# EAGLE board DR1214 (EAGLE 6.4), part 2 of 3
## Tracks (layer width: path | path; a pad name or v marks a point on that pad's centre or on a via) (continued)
GND  (via drill 0.15 layers 1-2, 0.15 layers 15-16, 0.25, 0.25 layers 2-15) (continued)
  other vias: 78.6,20.35 96.1,22.8 89.1,26 92.2,24.8 102,20.8 70,30 64.2,33.8 46.8,18.5 22.2,1.2 12.4,1.6 19.2,1.6 27.5,1.15 32,1.2 35.2,1.2 44,1.2 48.8,1.2 59.2,1.2 65.6,1.2 71.2,1.2 77.6,1.6 83.2,1.6 86,8.8 86.4,4 93.6,8.8 98.4,10.8 106.4,12.8 106.4,18.4 106.4,24.8 106.4,30.4 106.4,37.6 97.6,47.2 106.4,50 106.4,46.4 98.4,54 96,58.4 96,64 89.6,64 81.6,64 74.4,64 66.4,64 60,64 52.8,64 48,64 40.8,64 33.6,64 12.8,64 19.2,64 26.4,64 11.2,56 9.6,54.4 3.2,52.8 3.2,46.4 1.6,34.4 1.6,32 1.6,20.8 1.6,14 10.4,10.2 12.2,5.6 11.8,38 12.8,38.4 12.8,39.2 12.6,25.8 12.8,37.6 10.6,36 10.6,34.8 11.4,35.2 11.8,33.6 10.6,33.2 11.8,25 12.6,25 12.6,24.2 10.6,23 14.6,21.2 11.4,22.2 9.4,18.8 8.8,20.6 23.8,22.4 28,20 26,16.8 59.2,3.6 64.6,3.6 76.8,5.6 50.6,3.6 35.9,4.6 32.5,4.6 28,8 29.4,4.6 27.2,12.8 23,12.8 16.4,21.2 18,23.6 14.6,23.6 76.8,46 33,13 40.2,16 41.75,9.85 41.8,14.4 36,23.2 38.4,23.2 45,25.8 53.65,22.4 59,21 60.2,21.8 62.4,18.4 66.4,16 51.35,16.85 58.4,15.2 48.3,7.6 65.2,13.2 66,11.6 71.8,11.6 71.6,15.2 74.8,12.8 80,8 80.8,10.4 87.4,10.4 93.6,10.4 96,15.2 96,25.6 98.4,23.2 94.4,29.6 81.6,29.6 76.8,29.6 78.4,24.8 74.4,24.8 62.8,24 51.4,33.8 53.8,33.8 46.6,41.8 49.4,41.8 49.4,46.6 50.2,49 55.8,49.8 57.4,49.8 66,50 63.6,42 64.45,46.8 60.4,48.4 73.4,43.6 70.8,52 74.8,55.2 86.8,55.2 92.4,52.8 93.2,48.8 93.2,44.8 92.4,38.4 94.8,34.4 85.4,37.2 100.4,34.4 100.4,41.6 83.8,51.2 84.1,47.2 88,45.6 87.2,42.4 67.6,49.6 74.4,30.4 66,33.6 69.6,36.8 61.6,36 60,28 38.6,42.6 33,43.4 32.8,50.4 36.8,50.4 40,54.4 47.2,54.4 47.2,51.2 49.6,54.4 49.6,51.2 60.8,55.2 63.2,53.6 60.8,52 58,58.4 31.2,60 21.6,56.8 20,53.6 20.8,44.8 9.6,45.6 10.8,16 31.4,8.8 44.8,5.7 47,47.4 48,34 48,35.4 48,31.2 48,29.6 46.8,22.4 48,26.4 66.4,24 74.4,23.2 86.4,34.4 90.8,31.2 90.2,42 89.2,57.6 82.8,57.6 76.4,57.6 34.2,20.2 83.8,43.2 60.4,28.4 44.8,40.2 80.9,24.75 86.75,19.9 87.45,19.9 88.15,19.9 88.85,19.9 89.55,19.9 86.75,17.95 87.45,17.95 88.15,17.95 88.85,17.95 89.55,17.95 83.7,13.4 83.7,12.6 83.6,11.6 86,10.6 86.8,12.2 88,11.3 89.8,15.5 90.5,14.8 91.1,13.9 91.1,13.1 92.5,12.3 92.5,10.4 88.4,10.2 89.2,8.6 89.2,9.4 89.2,10.2 90.8,8.6 90.8,9.4 90.8,10.2 91.05,10.8 88.4,5 88.6,3.8 89.6,3 90.6,3 91.6,3.8 91.6,5 91.6,14.6 92,16.7 95.1,18.4 94.4,22.6 94.4,23.3 96,21.2 96,19 81.6,13.9 79.4,15.4 80.2,14.4 80,18.3 78.8,19.2 78.4,23.8 78.4,25.8 79.2,28.8 79.4,28 83,28.8 84.2,28.8 95.2,28.8 91.8,26.4 95.4,28 96,24.2 86.8,25 88.8,28.8 83.8,23 82,27 86.75,18.6 87.45,18.6 88.15,18.6 88.85,18.6 89.55,18.6 86.75,19.25 87.45,19.25 88.15,19.25 88.85,19.25 89.55,19.25 86.7,20.55 87.4,20.55 88.1,20.55 88.8,20.55 89.5,20.55 45,18.45 61.6,42.6 55.2,12.8 56.8,12.8 56.8,11.2 55.2,11.2 44.4,53.6 61.8,40 68.2,41.4 64.8,40.8 70.4,39.8 72,36.8 71.6,30.8 72.8,26.4 69.6,25.6 64.8,25.6 64.8,28.8 60.8,26.4 58.8,30 54,31.6 53.6,36 54.8,37.2 54.8,41.2 67.8,44 78.6,43.8 78.2,40 73.6,39.6 73,41.2 83.6,36.4 82.8,39.6 93.6,20 84.8,20 35.8,32.8 40.4,32.8 41.2,25.6 44.6,10.6 44.2,49.8 44.2,51.4 44.2,52.8 43.6,47 43.6,45.8 69,62.4 69,61.4 69,60.2 68.2,57 68.2,55.8 71.4,61.4 69.2,57 20,26.2 20,27.2 20,28.6 20.6,31.6 20.8,33.2 17.4,33.8 17.4,35.6 15.8,42.8 15.8,41.2 15.8,39.6 15.8,29 15.8,27.8 15.8,26.6 23.4,20.8 20.7,21.2 20.65,16.6 19.6,32.8 2.8,33.4 2.8,32.4 5,33.4 5,32.4 5,20.6 5,19.6 2.8,19.6 2.8,20.6 50.4,16.35 49.75,10.8 62.4,6.8 56.6,19.6 59.6,18.6 59.8,7.6 79.4,4 28,35.2 27,33.6 27,31.6 45.8,23.6 45.8,24.8 45.4,28.4 43.4,33.4 37,37 41.8,37 34.2,36.6 39.6,23.6 47.4,1.2 50.6,2.2 42.8,4 91,19.8 90.4,17.2 91.6,43.8 62.8,26 68,26 57,31.6 42.8,43.8 58.4,9.8 37.2,32.8 89.2,7.8 89.2,7 90.8,7.8 90.8,7 89.2,6.2 90.8,6.2 85,12.6 86.8,26.6 84.6,26.4 82.8,25.8 83.4,24.4 89.2,12.2 87.95,12.2 86.8,11.3 77.2,41.2 80,36.8 80,33.6 7.6,25.2 7.2,27.8 7.2,30.4 7.6,38.2 7.2,40 7.2,43 19.8,23.4 19.8,15 88.4,9.4 91.05,11.5 90.95,12.2 82.7,12 80.6,12.9 80.5,11.6 79.2,12.7 79.5,16.9 83,23 79.7,22.1 79.8,24.1 83.7,21.9 93.4,23.9 94.7,14.8 93.5,13.9 95.1,19.6 95.2,21.7 75.2,34.4 74.4,29.6 70.4,37.6 58.4,46.4 65.6,42.4 76.8,54.6 78.4,54.6 94,51.2 93,47.2 80.2,38.8 66.4,48.4 66.6,44 84.4,12.6 83.6,10.6 52.2,13.2 72,47.6 72,46 79.2,47.6 71.6,46.8 79.4,46.8 78.6,47.6 69.6,49.6 81.2,49.6 83.2,49.6 70.6,44 81.4,44 20.65,17.7 23.4,21.6 22.6,23.2 21.8,23.2 36.85,19.55 22.25,15.55 21.05,14.6 23.6,19.9 89.25,11.3 100.4,24 100.4,31.2
  pour Top (isolate 0.2, rank 6): 0,65 108,65 108,10.2 94.4,10.2 94.4,0 49.6,0 49.6,17.6 42.4,17.6 42.4,0 39.7,0 39.7,19.35 22.65,19.35 22.65,0 0,0
  pour Route3 (isolate 0.2): 0,64.8 108,64.8 108,10.2 94.4,10.2 94.4,0 0,0
  pour Bottom (isolate 0.2): 0,0 94.4,0 94.4,10.2 108,10.2 108,64.8 0,64.8
  pour Route15 (isolate 0.2): 0,0 94.4,0 94.4,10.2 108,10.2 108,64.8 0,64.8
  pour Route14 (isolate 0.2, rank 2): 0,0 94.4,0 94.4,10.2 108,10.2 108,64.8 0,64.8
  pour Route2 (isolate 0.2, rank 2): 0,0 94.4,0 94.4,10.2 108,10.2 108,64.8 0,64.8
GPI_0  (via drill 0.15 pad 0.1 layers 1-2, 0.25, 0.25 layers 2-15)
  Top 0.127: IC7.C16 | IC7.C16 v60.8,28.8
  Route2 0.127: v60.8,28.8 60.4,29.2 60.4,30.6 60.2,30.8 59.8,30.8 59.4,30.4 v57.2,30.4
  Route3 0.127: v48.8,30.4 48.8,55.6 50,56.8 53.6,56.8 55.2,58.4 v55.2,59.6
  Route14 0.127: v57.2,30.4 v48.8,30.4
  Bottom 0.127: v55.2,59.6 56.41,59.6 R131.1
  Bottom 0.305: R131.1 56.48,59.74 C104.1 54.49,61.65 BUT1.2
GPI_01/!SERVICE  (via drill 0.15 pad 0.1 layers 1-2, 0.25, 0.25 layers 2-15)
  Top 0.127: IC7.C15 v61.6,28.8 | PROG.2 32.25,43.45 v32.2,43.4
  Route2 0.127: v61.6,28.8 60.4,27.6 60.4,27 60.2,26.8 v55.6,26.8
  Route3 0.127: v47.2,39.6 v47.2,26.8
  Route14 0.127: v32.2,43.4 32.2,42 32.6,41.6 40.2,41.6 42.2,39.6 v47.2,39.6 | v55.6,26.8 v47.2,26.8
  Bottom 0.254: R61.1 28.34,45.73 28,45.4 28,43.6 28.6,43 31.8,43 v32.2,43.4
  Bottom 0.406: R62.2 R61.1
GPI_4  (via drill 0.15 pad 0.1 layers 1-2, 0.25, 0.25 layers 2-15)
  Top 0.127: IC7.E13 v62.4,29.6
  Route2 0.127: v62.4,29.6 62,29.2 62,26.2 61,25.2 v57.6,25.2
  Route3 0.127: v48.4,25.2 48.4,59.6 v48,60
  Route14 0.127: v57.6,25.2 v48.4,25.2
  Bottom 0.127: v48,60 47.01,60 R132.1
  Bottom 0.305: R132.1 C105.1 BUT2.2
GPIO_00  (via drill 0.15 layers 1-2, 0.15 pad 0.1 layers 1-2, 0.25 layers 2-15, 0.25 pad 0.1 layers 2-15)
  Top 0.127: v90.4,26 90.4,25.25 R138.1 | IC7.A12 v63.61,26.21 v63.6,26.2
  Route2 0.127: v63.6,26.2 v63.6,26.8 | v91.4,24.8 91.4,25 v90.4,26
  Route14 0.127: v63.6,26.8 64.4,26 73.2,26 74,25.2 80.8,25.2 81.2,25.6 90.6,25.6 v91.4,24.8
GPIO_01  (via drill 0.15 pad 0.1 layers 1-2, 0.25, 0.25 layers 2-15)
  Top 0.127: EXT.12 73.2,7.58 v73.2,9.2 | IC7.A11 v64.4,26.2
  Route2 0.127: v64.4,26.2 v64.4,19.6
  Route14 0.127: v64.4,19.6 64.6,19.6 65.4,18.8 71.4,18.8 72,18.2 72,12.2 73.2,11 v73.2,9.2
GPIO_04/SSEL1/LCDVD[22]  (via drill 0.15 pad 0.1 layers 1-2, 0.25, 0.25 layers 2-15)
  Top 0.127: IC7.B11 64.4,27.6 v64,27.2 | 68.2,3.71 EXT.3 v68.19,5.39 v68.2,5.4
  Route2 0.127: v64,27.2 64,18.8 v63.6,18.4
  Route14 0.127: v63.6,18.4 64.4,17.6 67.2,17.6 68,16.8 68,5.6 v68.2,5.4
GPO19/!WP_NAND  (via drill 0.15 layers 15-16, 0.15 pad 0.1 layers 1-2, 0.25 layers 2-15)
  Top 0.127: IC7.C2 v72.8,27.2
  Route2 0.127: v72.8,27.2 72.8,22.8 v73.6,22
  Route3 0.127: v85.2,17.8 84.6,17.8 83.8,18.6 82,18.6 78.6,22 v77.2,22
  Route14 0.127: v73.6,22 v77.2,22
  Route15 0.127: v85.8,17.8 v85.2,17.8
  Bottom 0.127: v85.8,17.8 86.7,17.8 R79.1
GPO_01  (via drill 0.15 layers 1-2, 0.25, 0.25 layers 2-15)
  Top 0.127: IC7.D4 v70.4,29.6
  Route2 0.127: v70.4,29.6 70.4,28.8 70,28.4 v70,23.2
  Route3 0.127: v40.4,40 v40.4,23.2 | v56.8,23.2 v61.2,23.2 | v27.8,56.2 29,56.2 31.2,54 31.2,51.6 v30.6,51
  Route14 0.127: v40.4,40 39.6,40.8 32,40.8 30.4,42.4 30.4,50.8 v30.6,51 | v40.4,23.2 v56.8,23.2 | v70,23.2 v61.2,23.2
  Bottom 0.127: R63.2 27.94,56.34 v27.8,56.2
GPO_02  (via drill 0.15 pad 0.1 layers 1-2, 0.25, 0.25 layers 2-15)
  Top 0.127: IC7.B14 v61.6,27.2
  Route2 0.127: v61.6,27.2 60.4,26 v56.8,26
  Route3 0.127: v22.8,56.2 22.8,55.6 23.2,55.2 26.8,55.2 v30,52 | v40,39.6 v40,22.4 | v46,22.4 v46,26
  Route14 0.127: v30,52 30,42.2 31.8,40.4 39.2,40.4 v40,39.6 | v40,22.4 v46,22.4 | v56.8,26 v46,26
  Bottom 0.127: R64.2 22.86,56.26 v22.8,56.2
GPO_03  (via drill 0.15 pad 0.1 layers 1-2, 0.25, 0.25 layers 2-15)
  Top 0.127: IC7.D12 v63.2,28.8
  Route2 0.127: v63.2,28.8 62.4,28 62.4,26 61.2,24.8 v55.2,24.8
  Route3 0.127: v17.8,56.2 17.8,55.6 18.6,54.8 26.4,54.8 v29.4,51.8 | v38.8,40 39.6,39.2 v39.6,24.4
  Route14 0.127: v29.4,51.8 29.6,51.6 29.6,42 31.6,40 v38.8,40 | v39.6,24.4 45.8,24.4 46.2,24.8 v55.2,24.8
  Bottom 0.127: R65.2 17.78,56.22 v17.8,56.2
GPO_04  (via drill 0.15 layers 1-2, 0.25 layers 2-15)
  Top 0.127: IC7.D8 v67.2,28.8
  Top 0.15: v78.2,26.4 79,26.4 D3.3
  Route2 0.127: v67.2,28.8 v67.2,28 | v77.6,26.4 v78.2,26.4
  Route14 0.127: v67.2,28 68,27.2 73.8,27.2 74.6,26.4 v77.6,26.4
GPO_05  (via drill 0.15 layers 1-2, 0.15 pad 0.1 layers 1-2, 0.25 layers 2-15)
  Top 0.127: IC7.B3 v71.2,27.2
  Top 0.254: D4.3 94.68,17.62 v94.6,17.7
  Route2 0.127: v71.2,27.2 71.6,26.8 v71.6,22.4 | v94,17.7 v94.6,17.7
  Route3 0.127: v77.8,22.4 78.8,22.4 82.2,19 92.7,19 v94,17.7
  Route14 0.127: v71.6,22.4 v77.8,22.4
GPO_14  (via drill 0.15 layers 1-2, 0.25, 0.25 layers 2-15)
  Top 0.127: IC7.D3 v71.2,28.8
  Route2 0.127: v72.4,23.6 72.4,27.6 v71.2,28.8
  Route3 0.127: v40.8,40.4 v40.8,23.6 | v57.6,23.6 v60.6,23.6 | v31,50.6 31.6,51.2 31.6,54.8 v33,56.2
  Route14 0.127: v40.8,40.4 40,41.2 32.2,41.2 30.8,42.6 30.8,50.4 v31,50.6 | v72.4,23.6 v60.6,23.6 | v40.8,23.6 v57.6,23.6
  Bottom 0.127: R3.2 33.02,56.22 v33,56.2
GPO_23/U2_HRTS/U3_RTS  (via drill 0.15 layers 1-2, 0.25, 0.25 layers 2-15)
  Top 0.127: IC7.M16 v60,35.2 | v69.4,9.2 69.4,7.57 EXT.6
  Route2 0.127: v60,35.2 59.6,35.2 59.2,35.6 v54.8,35.6
  Route3 0.127: v54.8,35.6 54.8,33.6 53.4,32.2 53.4,23.6 63,14 v68.8,14
  Route14 0.127: v68.8,14 68.8,9.8 v69.4,9.2
I2C1_SCL  (via drill 0.15 pad 0.1 layers 1-2, 0.25, 0.25 layers 2-15)
  Top 0.127: IC7.A5 v69.2,26.2
  Route2 0.127: v69.2,26.2 69.2,23 69.6,22.6 69.6,22 v70,21.6
  Route14 0.127: v70,21.6 71.6,21.6 74,19.2 74,15.4 v74.6,14.8
  Bottom 0.127: v74.6,14.8 75.95,14.8 IC4.6
  Bottom 0.254: IC4.6 79.33,14.68 80.5,13.5 80.5,12.85
  Bottom 0.305: 80.5,12.85 R71.1
I2C1_SDA  (via drill 0.15 pad 0.1 layers 1-2, 0.25, 0.25 layers 2-15)
  Top 0.127: IC7.B6 68.39,27.61 v68.8,27.2
  Route2 0.127: v68.8,27.2 68.4,26.8 68.4,21.8 v69.2,21
  Route14 0.127: v69.2,21 71.6,21 73.6,19 73.6,15 v74.6,14
  Bottom 0.127: v74.6,14 76.05,14 IC4.5
  Bottom 0.254: IC4.5 76.08,12.78
  Bottom 0.305: 76.08,12.78 R72.1
I2C2_SCL  (via drill 0.15 pad 0.1 layers 1-2, 0.25, 0.25 layers 2-15)
  Top 0.127: IC7.A3 v71.2,26.4 | v65.6,7.2 65.91,7.5 EXT.2 67,7.58 v67,9.2
  Route2 0.127: v71.2,26.4 v71.2,18.4
  Route3 0.127: v70.4,13.2 v67,13.2
  Route14 0.127: v71.2,18.4 70.6,18.4 70.4,18.2 v70.4,13.2 | v67,13.2 v67,9.2
  Bottom 0.127: R73.1 65.45,7.05 v65.6,7.2
I2C2_SDA  (via drill 0.15 pad 0.1 layers 1-2, 0.25, 0.25 layers 2-15)
  Top 0.127: IC7.E4 70.01,30.01 v70.4,30.4 | EXT.1 67,3.77 v67,5.4
  Route2 0.127: v70.4,30.4 70.8,30 v70.8,17.8
  Route3 0.127: v70.8,12.8 v67.4,12.8
  Route14 0.127: v70.8,17.8 v70.8,12.8 | v67.4,12.8 67.4,5.8 v67,5.4
  Bottom 0.127: R74.1 66.3,4.7 v67,5.4
J_RX1  (via drill 0.25, 0.38)
  Top 0.254: IC11.40 85.87,23.33 v85.6,23.6 | JUART1.2 103.45,25.2 v103.3,25.35
  Route3 0.254: v85.6,23.6 86.2,24.2 89,24.2 91.6,26.8 101.85,26.8 v103.3,25.35
J_TX1  (via drill 0.25, 0.38)
  Top 0.254: IC11.38 86.87,23.33 v86.6,23.6 | JUART1.1 104.83,23.23 v104.8,23.2
  Route3 0.254: v86.6,23.6 89.2,23.6 91.8,26.2 101.25,26.2 104.25,23.2 v104.8,23.2
J_VDD  (via drill 0.15 layers 1-2, 0.25, 0.25 layers 2-15)
  Top 0.254: IC11.9 84.64,17.49 v84.45,17.3 83.2,16.05 C108.1 | IC11.30 91.04,21.49 91.04,22.29 v91.15,22.4 91.55,22.8 C109.1
  Top 0.406: C110.1 85.65,25.4 | 85.65,25.4 L11.1 | 85.65,25.4 85.65,25.25 84.6,24.2 v84.6,22.4
  Route2 0.254: v91.15,22.4 v90.4,22.4 | v84.6,18.5 84.6,17.45 v84.45,17.3
  Route14 0.406: v90.4,22.4 v84.6,22.4 v84.6,18.5
JTAG_NTRST  (via drill 0.15 pad 0.1 layers 1-2, 0.25, 0.25 layers 2-15)
  Top 0.127: IC7.H17 59.6,32.4 v59.2,32.8
  Route2 0.127: v59.2,32.8 58.8,33.2 v57.6,33.2
  Route3 0.127: v46,33.2 v46,39.2
  Route14 0.127: v57.6,33.2 v46,33.2 | v46,39.2 31.2,39.2 28.8,41.6 28.8,50 v28.4,50.4
  Bottom 0.127: v28.4,50.4 28.6,50.6 29.8,50.6 29.95,50.75 D10.1 29.95,53.8 R18.1
JTAG_RTCK  (via drill 0.25, 0.25 layers 2-15)
  Top 0.254: JTAG.7 19.33,47.93 v19.4,48
  Route3 0.127: v45.6,32.8 v45.6,38
  Route14 0.127: v52.4,32.8 v45.6,32.8 | v45.6,38 30.6,38 27.6,41 27.6,47.6 26.8,48.4 25.4,48.4 24.4,47.4 22.8,47.4 21.6,48.6 20,48.6 v19.4,48
  Bottom 0.127: R110.2 v52.4,32.8
  Bottom 0.254: R22.1 17.25,46.7 R29.2 19.4,47.5 v19.4,48
JTAG_TCK  (via drill 0.15 layers 1-2, 0.25, 0.25 layers 2-15)
  Top 0.127: v62.4,32.8 v62.4,32.79 IC7.H14
  Top 0.254: JTAG.4 23.13,50.47 v23.2,50.4
  Route2 0.127: v56.4,35.2 59,35.2 59.4,34.8 61.4,34.8 62.4,33.8 v62.4,32.8
  Route3 0.127: v50.4,37.6 v50.4,35.2 | v26.8,47.6 26.4,47.2 25.6,47.2 25.2,47.6 25.2,49.4 24.2,50.4 v23.2,50.4
  Route14 0.127: v50.4,37.6 30.4,37.6 27.2,40.8 27.2,47.2 v26.8,47.6 | v50.4,35.2 v56.4,35.2
  Bottom 0.254: v23.2,50.4 R24.2
JTAG_TDI  (via drill 0.15 pad 0.1 layers 1-2, 0.25, 0.25 layers 2-15)
  Top 0.127: IC7.J16 60.4,33.2 v60,33.6
  Top 0.254: JTAG.8 23.13,47.93 v23.2,48
  Route2 0.127: v60,33.6 59.8,33.6 59,34.4 v56.4,34.4
  Route3 0.127: v46.4,34.4 v46.4,38.4
  Route14 0.127: v56.4,34.4 v46.4,34.4 | v46.4,38.4 30.8,38.4 28,41.2 28,47.8 27,48.8 25.2,48.8 24.4,48 v23.2,48
  Bottom 0.254: R20.1 23.4,47.8 v23.2,48
JTAG_TDO  (via drill 0.25, 0.25 layers 2-15)
  Top 0.254: JTAG.6 v23.2,49.2
  Route3 0.127: v46.8,34.8 v46.8,38.8
  Route14 0.127: v52.4,34.8 v46.8,34.8 | v46.8,38.8 31,38.8 28.4,41.4 28.4,48 27.2,49.2 v23.2,49.2
  Bottom 0.127: R111.2 v52.4,34.8
  Bottom 0.254: R23.1 v23.2,49.2
JTAG_TMS  (via drill 0.15 pad 0.1 layers 1-2, 0.25, 0.25 layers 2-15)
  Top 0.127: IC7.G18 v59.2,32 | v23.2,51.8 21.36,51.8 JTAG.2
  Top 0.254: JTAG.2 21.3,53.45 v21.15,53.6
  Route2 0.127: v59.2,32 v56,32
  Route3 0.127: v44.8,37.2 v44.8,32 | v25.8,47.8 25.8,49.4 23.4,51.8 v23.2,51.8
  Route14 0.127: v25.8,47.8 26.8,46.8 26.8,40.6 30.2,37.2 v44.8,37.2 | v56,32 v44.8,32
  Bottom 0.254: R21.1 23.4,51.6 v23.2,51.8
LINK/ACT  (via drill 0.25)
  Route3 0.254: v34.95,31.85 35,31.8 35,19.8 41,13.8 41,6.74 ETH.C2
  Bottom 0.254: U201.22 35.62,31.18 v34.95,31.85 | R28.2 37.88,3.7 ETH.C2
N$1
  Bottom 0.254: U201.28 38.62,32.42 39.6,33.4 39.6,34 Q201.4
  Bottom 0.305: R40.2 40.1,34.6 Q201.4
N$2
  Bottom 0.254: IC1.2 32.7,49.3 31.8,50.2 30.92,50.2 D10.3
  Bottom 0.406: IC1.2 32.95,47.84 IC2.1
N$3  (via drill 0.25)
  Top 0.254: LED1.A 38.89,59.15 v38.1,59.94
  Bottom 0.305: v38.1,59.94 R2.1
N$4  (via drill 0.25)
  Top 0.254: LED2.A 33.81,59.15 v33.02,59.94
  Bottom 0.305: v33.02,59.94 R3.1
N$5  (via drill 0.15 layers 15-16)
  other vias: 38.8,27.9
N$6
  Bottom 0.254: U201.20 34.37,30.13 34,30.5 32.65,30.5 R4.1
N$7
  Bottom 0.61: L15.1 45.35,9.38 USB.1
N$8
  Top 0.254: R148.2 54.5,9.75 IC13.19
N$9  (via drill 0.15 layers 1-2, 0.25)
  Top 0.127: IC7.N13 62.81,36.41 v63.2,36.8 IC7.N12
  Route2 0.127: v63.2,36.8 v63.2,41.2
  Bottom 0.127: v63.2,41.2 C41.1
  Bottom 0.305: L1.2 61.8,42.85 C42.1 61.75,41.5 C41.1
N$10
  Top 0.254: IC13.18 52.45,10.75 R30.2
N$11
  Top 0.254: IC13.6 58.5,13.25 59.55,14.3 R16.1 R15.2
N$12
  Top 0.5: RF.1 90,13.27 L13.2
N$13
  Top 0.305: IC5.8 R36.2
N$14
  Top 0.254: IC13.8 56.75,16.35 R19.2
  Top 0.305: R19.2 R17.1
N$15  (via drill 0.15 layers 15-16)
  other vias: 37.4,26.7
N$16
  Top 0.305: IC5.2 9,23.23 8.23,24 C10.1
N$17
  Top 0.813: DC-IN.3 13.53,13.47 12,15 12,17.39 D6.A
  Bottom 0.406: C21.1 13.63,11.25 DC-IN.3
N$18  (via drill 0.15 pad 0.1 layers 1-2)
  Top 0.127: IC7.R14 v61.6,37.6 | C65.2 R55.2 53.85,39.2 v54.8,39.2
  Route2 0.127: v61.6,37.6 61.6,38.4 60.8,39.2 v54.8,39.2
N$19  (via drill 0.15 layers 15-16)
  other vias: 37.4,27.9
N$20
  Bottom 0.254: U201.18 32.87,29.13 32.75,29.25
  Bottom 0.406: 29.35,29.25 31,29.25 | 31,29.25 32.75,29.25 | C137.1 29.5,29.4 29.35,29.25 | 31,29.25 C134.1 | 29.35,29.25 28.35,29.25 L17.1
N$21  (via drill 0.15 layers 1-2, 0.25)
  Top 0.127: IC7.P13 v62.4,37.6
  Route2 0.127: v62.4,37.6 62.4,39.6 61.2,40.8 v58.4,40.8
  Bottom 0.127: v58.4,40.8 59.75,40.8 C41.2
  Bottom 0.305: L2.2 59.6,43.05 C42.2 59.85,41.5 C41.2
N$22  (via drill 0.15 layers 1-2, 0.15 layers 15-16, 0.25 layers 2-15)
  Top 0.127: IC7.N14 v61.6,36.8
  Route2 0.127: v61.6,36.8 v62,36.4
  Route15 0.127: v62,36.4 v61.6,36.8
  Bottom 0.127: R46.1 61.4,36.6 v61.6,36.8
N$23  (via drill 0.15 layers 1-2, 0.25, 0.25 layers 2-15)
  Top 0.127: IC7.G14 61.6,31.2 v60.8,31.2
  Route2 0.127: v60.8,31.2 v55.2,31.2
  Route3 0.127: v50,31.2 v50,43.4
  Route14 0.127: v55.2,31.2 v50,31.2
  Bottom 0.127: v50,43.4 R135.2 R12.2
N$24  (via drill 0.15 layers 1-2, 0.15 layers 15-16, 0.25 layers 2-15)
  Top 0.127: IC7.K14 61.6,34.4 v61.6,35.2
  Route2 0.127: v61.6,35.2 v61.2,35.6
  Route15 0.127: v61.2,35.6 v61.6,35.2
  Bottom 0.127: R48.1 C45.1 61.4,35.4 v61.6,35.2 61.8,35.4 R47.1
N$25
  Top 0.254: C63.2 50.2,38.72 Q4.1 52.7,38.12 R49.1
N$26
  Top 0.254: Q5.1 55.6,48 56.2,47.4 56.35,47.4 C61.2 56.6,46.75 56.6,45.6 56.4,45.4 55.6,45.4 55.4,45.2 55.4,44.85 R53.1
N$27  (via drill 0.5)
  Top 0.406: v21.43,25.22 21.43,26.46 U4.4 | C2.2 R13.1 v21.43,34.42 R14.2 C19.1
  Route3 0.406: v21.43,34.42 v21.43,25.22
N$28
  Top 0.61: U4.5 22.57,28.39 L7.P$1
N$29
  Top 0.406: 24.04,35.75 25.52,35.75 LR8.1
  Top 0.61: L7.P$2 26,29.53 25.24,30.3 C5.1 C3.1 23.98,32.95 R13.2 C2.1 24.04,35.75
N$30
  Top 0.254: 52.8,46.2 52.15,46.2 C60.2
  Top 0.305: R54.1 52.8,46.2 Q5.3
N$31
  Bottom 0.254: R25.2 24.43,5.7 ETH.A1
N$32
  Bottom 0.2: L6.1 35.17,34.68 C141.1 36.82,34.68 Q201.6
N$34
  Top 0.254: C62.2 49.76,34.38 | 49.76,34.38 49.78,34.38 50.8,35.4 Q4.2 52.44,35.62 R52.1 | C20.1 50.25,33.89 49.76,34.38
N$35  (via drill 0.15 pad 0.1 layers 1-2)
  Top 0.127: IC7.P17 v59.2,37.6 | R49.2 54.4,37.8 v55,38.4
  Route2 0.127: v59.2,37.6 58.4,38.4 v55,38.4
N$36
  cutout Route2: 84,16 91.2,16 91.2,10.8 90.45,10.8 90.45,4 89.55,4 89.55,10.8 84,10.8
N$37
  Bottom 0.127: R86.2 71.4,46.2 71.6,46.4 79.4,46.4 79.6,46.2 R38.1
N$38  (via drill 0.15 pad 0.1 layers 1-2)
  Top 0.127: IC7.P16 60.39,37.19 v60,36.8 | v55.4,36.4 55.2,36.4 55,36.2 R52.2
  Route2 0.127: v60,36.8 59.6,37.2 59,37.2 58.2,38 55.6,38 55.4,37.8 v55.4,36.4
N$39
  Bottom 0.254: R27.2 37.81,5.7 ETH.A2
N$40
  Bottom 0.127: R87.2 71.4,47.4 71.6,47.2 79.4,47.2 79.6,47.4 R39.1
N$41
  Top 0.127: IC7.R15 60.8,38.4 60.8,39 60.6,39.2 59.4,39.2 59,39.6 58,39.6 55.2,42.4 R53.2
N$42
  Top 0.127: IC7.T17 59.42,38.78 59,39.2 57.8,39.2 54.8,42.2 53,42.2 52.8,42.4 R54.2
N$43
  Top 0.127: 50.45,39.6 C64.2
  Top 0.254: 50.45,39.6 R55.1
N$45  (via drill 0.15 layers 1-2, 0.25)
  Top 0.127: IC7.M14 62.01,35.61 v62.4,36
  Route2 0.127: v62.4,36 62.8,36.4 62.8,39.8 61.4,41.2 58.8,41.2 v57.6,42.4
  Bottom 0.127: R56.1 57.4,42.6 v57.6,42.4
  Bottom 0.254: R56.1 53.05,43.45 IC8.4
N$46  (via drill 0.25)
  Top 0.254: LED3.A 28.73,59.15 v27.94,59.94
  Bottom 0.305: v27.94,59.94 R63.1
N$50  (via drill 0.25)
  Top 0.254: LED4.A 23.65,59.15 v22.86,59.94
  Bottom 0.305: v22.86,59.94 R64.1
N$52  (via drill 0.25)
  Top 0.254: LED5.A 18.57,59.15 v17.78,59.94
  Bottom 0.305: v17.78,59.94 R65.1
N$54
  Top 0.254: R140.1 83.1,13.25 83.1,13.5 83.9,14.3 83.9,15.64 IC11.10
N$55
  Top 0.254: IC11.4 84.11,19.99 83.5,20.6 81.4,20.6 81.1,20.9 81.1,21.6 Q12.1 81.05,21.75 C106.2
N$58  (via drill 0.15 pad 0.1 layers 1-2, 0.25 layers 2-15, 0.25 pad 0.1)
  Top 0.127: IC7.G2 71.61,31.61 v72,32
  Route2 0.127: v72,32 74.8,32 v75.2,31.6
  Route14 0.127: v75.2,31.6 88.6,31.6 94.6,37.6 v94.6,39.2
  Bottom 0.127: IC9.42 94.75,39.35 v94.6,39.2
N$59  (via drill 0.15 pad 0.1 layers 1-2, 0.25 layers 2-15, 0.25 pad 0.1)
  Top 0.127: IC7.G3 70.81,31.61 v71.2,32
  Route2 0.127: v71.2,32 71.6,32.4 75.6,32.4 v76.8,31.2
  Route14 0.127: v76.8,31.2 88.8,31.2 95.2,37.6 v95.2,38.2
  Bottom 0.127: IC9.43 95.25,38.25 v95.2,38.2
N$60  (via drill 0.15 pad 0.1 layers 1-2, 0.25 layers 2-15, 0.25 pad 0.1)
  Top 0.127: IC7.H2 71.6,32.4 v72,32.8
  Route2 0.127: v72,32.8 v73.4,32.8
  Route14 0.127: v73.4,32.8 74.2,33.6 87.6,33.6 88,34 v88,37.6
  Bottom 0.127: IC9.29 88.25,37.85 v88,37.6
N$61  (via drill 0.15 pad 0.1 layers 1-2, 0.25 layers 2-15, 0.25 pad 0.1)
  Top 0.127: IC7.H3 70.8,32.4 v71.2,32.8
  Route2 0.127: v71.2,32.8 71.6,33.2 v74.8,33.2
  Route14 0.127: v74.8,33.2 87.8,33.2 88.6,34 v88.6,37.6
  Bottom 0.127: IC9.30 88.8,40.58 88.8,37.8 v88.6,37.6
N$62  (via drill 0.15 pad 0.1 layers 1-2, 0.25 layers 2-15, 0.25 pad 0.1)
  Top 0.127: IC7.F1 72.41,30.81 v72.8,31.2
  Route2 0.127: v72.8,31.2 v73.6,31.2
  Route14 0.127: v73.6,31.2 73.6,31.8 74.2,32.4 76.6,32.4 77,32.8 88,32.8 89.2,34 v89.2,38.6
  Bottom 0.127: IC9.31 89.25,38.65 v89.2,38.6
N$63  (via drill 0.15 pad 0.1 layers 1-2, 0.25 layers 2-15, 0.25 pad 0.1)
  Top 0.127: IC7.E1 72.41,30.01 v72.8,30.4
  Route2 0.127: v72.8,30.4 v73.6,30.4
  Route14 0.127: v73.6,30.4 74,30.8 74,31.6 74.4,32 76.8,32 77.2,32.4 88.2,32.4 89.8,34 v89.8,38.6
  Bottom 0.127: IC9.32 89.75,38.65 v89.8,38.6
N$64  (via drill 0.15 pad 0.1 layers 1-2, 0.25 layers 2-15, 0.25 pad 0.1)
  Top 0.127: 70,32.4 v70.4,32.8
  Top 0.254: IC7.H4 70,32.4
  Route2 0.127: v70.4,32.8 71.2,33.6 76,33.6 v77.6,32
  Route14 0.127: v77.6,32 88.4,32 94,37.6 v94,39.2
  Bottom 0.127: IC9.41 94.25,39.45 v94,39.2
N$65  (via drill 0.15 pad 0.1 layers 1-2, 0.25 layers 2-15, 0.25 pad 0.1)
  Top 0.127: IC7.E2 71.61,30.01 v72,30.4
  Route2 0.127: v72,30.4 72.4,30.8 74,30.8 v74.4,31.2
  Route14 0.127: v74.4,31.2 76.2,31.2 76.6,30.8 89,30.8 95.8,37.6 v95.8,38.2
  Bottom 0.127: IC9.44 95.75,38.25 v95.8,38.2
N$66  (via drill 0.15 pad 0.1 layers 1-2, 0.25 layers 2-15, 0.25 pad 0.1)
  Top 0.127: IC7.D2 v72,28.8
  Route2 0.127: v72,28.8 73.6,27.2 v75.6,27.2
  Route14 0.127: v75.6,27.2 89.8,27.2 90.2,27.6 v91,27.6
  Bottom 0.15: IC9.17 89.75,25.35 91,26.6 v91,27.6
N$67  (via drill 0.15 pad 0.1 layers 1-2, 0.25 layers 2-15, 0.25 pad 0.1)
  Top 0.127: IC7.E3 v71.2,29.6
  Route2 0.127: v71.2,29.6 71.6,29.2 73,29.2 73.8,28.4 v75.6,28.4
  Route14 0.127: v75.6,28.4 89.2,28.4 89.6,28.8 92.6,28.8 92.8,28.6 v92.8,28
  Bottom 0.127: IC9.9 93.75,27.05 v92.8,28
N$68  (via drill 0.15 pad 0.1 layers 1-2, 0.25 layers 2-15, 0.25 pad 0.1)
  Top 0.127: IC7.F2 71.61,30.81 v72,31.2
  Route2 0.127: v72,31.2 72.4,31.6 74.6,31.6 74.8,31.4 74.8,30.6 v75.6,29.8
  Route14 0.127: v75.6,29.8 74.8,29 74.8,27.2 75.2,26.8 90,26.8 v90.4,27.2
  Bottom 0.15: IC9.18 89.25,25.65 90.4,26.8 v90.4,27.2
N$69  (via drill 0.15 pad 0.1 layers 1-2, 0.25 layers 2-15, 0.25 pad 0.1)
  Top 0.127: IC7.C1 v72.8,28.8
  Route2 0.127: v72.8,28.8 73.6,28 v76.8,28
  Route14 0.127: v76.8,28 89.4,28 89.8,28.4 v92.2,28.4
  Bottom 0.127: IC9.8 94.25,27.15 93,28.4 v92.2,28.4
N$70  (via drill 0.15 pad 0.1 layers 1-2, 0.25 layers 2-15, 0.25 pad 0.1)
  Top 0.127: IC7.F3 70.81,30.81 v71.2,31.2
  Route2 0.127: v71.2,31.2 71.6,30.8 71.6,30.2 71.8,30 73.4,30 74.2,29.2 v75.6,29.2
  Route14 0.127: v75.6,29.2 75.2,28.8 75.2,27.8 75.4,27.6 89.6,27.6 90,28 91.6,28 v92.2,27.4
  Bottom 0.15: v92.2,27.4 92.2,27.2 90.25,25.25 IC9.16
N$71  (via drill 0.15 pad 0.1 layers 1-2, 0.25 layers 2-15, 0.25 pad 0.1)
  Top 0.127: IC7.D1 v72.8,29.6
  Route2 0.127: v72.8,29.6 73.2,29.6 74,28.8 v77.2,28.8
  Route14 0.127: v77.2,28.8 89,28.8 89.4,29.2 v93.2,29.2
  Bottom 0.127: IC9.7 94.75,27.25 93.2,28.8 v93.2,29.2
  Bottom 0.254: IC9.7 94.75,19.4
  Bottom 0.305: 94.75,19.4 R58.1
N$72
  Bottom 0.254: R79.2 R78.1 88.75,19.65 IC9.19
N$73
  Top 0.127: IC7.U16 60,40 60,43.2 58.25,44.95 C69.1
N$74
  Top 0.127: C70.1 63,43.8 62.8,43.6 62.8,41 63.2,40.6 63.2,38.4 62.81,38.01 IC7.R13
N$75
  Top 0.127: C71.1 59.4,44.4
  Top 0.15: IC7.V16 60.42,43.38 59.4,44.4
N$76
  Top 0.127: C72.1 61.8,43.8 62.4,43.2 62.4,39.2 62.01,38.81 IC7.T14
N$77
  Top 0.127: C73.1 60.6,43.8 60.8,43.6 60.8,39.99 IC7.U15
N$110  (via drill 0.25)
  Top 0.127: IC7.V8 66.8,42 v65.6,43.2
  Bottom 0.127: v65.6,43.2 R26.1
N$111  (via drill 0.25)
  Top 0.127: IC7.R9 65.6,38.4 65.6,40.8 v64.8,41.6
  Bottom 0.127: v64.8,41.6 64.8,43.95 R31.1
N$114  (via drill 0.15 layers 1-2)
  Top 0.127: IC7.T2 72,39.2 v72,40 | RN10.1 v74.6,43.4
  Route2 0.127: v74.6,43.4 74.4,43.4 73.8,42.8 73.8,41.6 72.2,40 v72,40
N$115
  Bottom 0.127: R82.1 69.6,44.95 arc-90 69.85,44.7 69.85,44.63 arc90 70.1,44.38 70.15,44.38 arc90 70.4,44.63 70.4,45.27 arc-90 70.65,45.52 70.69,45.52 arc-90 70.94,45.27 70.94,44.63 arc90 71.2,44.38 71.24,44.38 arc90 71.49,44.63 71.49,45.27 arc-90 71.75,45.52 71.79,45.52 arc-90 72.04,45.27 72.04,44.63 arc90 72.29,44.38 72.34,44.38 arc90 72.59,44.63 72.59,45.27 arc-90 72.84,45.52 72.88,45.52 arc-90 73.14,45.27 73.14,44.63 arc90 73.39,44.38 73.43,44.38 arc90 73.68,44.63 73.68,45.27 arc-90 73.94,45.52 73.98,45.52 arc-90 74.23,45.27 74.23,44.63 arc90 74.48,44.38 74.53,44.38 arc90 74.78,44.63 74.78,45.27 arc-90 75.03,45.52 75.07,45.52 arc-90 75.33,45.27 75.33,44.63 arc90 75.58,44.38 75.62,44.38 arc90 75.87,44.63 75.87,45.27 arc-90 76.12,45.52 76.17,45.52 arc-90 76.42,45.27 76.42,44.63 arc90 76.67,44.38 76.72,44.38 arc90 76.97,44.63 76.97,45.27 arc-90 77.22,45.52 77.26,45.52 arc-90 77.52,45.27 77.52,44.63 arc90 77.77,44.38 77.81,44.38 arc90 78.06,44.63 78.06,45.27 arc-90 78.31,45.52 78.36,45.52 arc-90 78.61,45.27 78.61,44.63 arc90 78.86,44.38 78.91,44.38 arc90 79.16,44.63 79.16,45.27 arc-90 79.41,45.52 79.45,45.52 arc-90 79.7,45.27 79.7,44.63 arc90 79.96,44.38 80,44.38 arc90 80.25,44.63 80.25,45.27 arc-90 80.5,45.52 80.55,45.52 arc-90 80.8,45.27 80.8,44.63 arc90 81.05,44.38 81.1,44.38 arc90 81.35,44.63 81.35,44.7 arc-90 81.6,44.95 R83.1
N$116
  Bottom 0.127: R84.1 69.44,48.65 arc-90 69.69,48.4 69.69,48.37 arc90 69.94,48.12 69.95,48.12 arc90 70.2,48.37 70.2,48.93 arc-90 70.45,49.18 70.45,49.18 arc-90 70.71,48.93 70.71,48.37 arc90 70.96,48.12 70.96,48.12 arc90 71.21,48.37 71.21,48.93 arc-90 71.47,49.18 71.47,49.18 arc-90 71.72,48.93 71.72,48.37 arc90 71.97,48.12 71.97,48.12 arc90 72.23,48.37 72.23,48.93 arc-90 72.48,49.18 72.48,49.18 arc-90 72.73,48.93 72.73,48.37 arc90 72.98,48.12 72.99,48.12 arc90 73.24,48.37 73.24,48.93 arc-90 73.49,49.18 73.5,49.18 arc-90 73.75,48.93 73.75,48.37 arc90 74,48.12 74,48.12 arc90 74.25,48.37 74.25,48.93 arc-90 74.51,49.18 74.51,49.18 arc-90 74.76,48.93 74.76,48.37 arc90 75.01,48.12 75.02,48.12 arc90 75.27,48.37 75.27,48.93 arc-90 75.52,49.18 75.52,49.18 arc-90 75.77,48.93 75.77,48.37 arc90 76.03,48.12 76.03,48.12 arc90 76.28,48.37 76.28,48.93 arc-90 76.53,49.18 76.53,49.18 arc-90 76.79,48.93 76.79,48.37 arc90 77.04,48.12 77.04,48.12 arc90 77.29,48.37 77.29,48.93 arc-90 77.55,49.18 77.55,49.18 arc-90 77.8,48.93 77.8,48.37 arc90 78.05,48.12 78.06,48.12 arc90 78.31,48.37 78.31,48.93 arc-90 78.56,49.18 78.56,49.18 arc-90 78.81,48.93 78.81,48.37 arc90 79.07,48.12 79.07,48.12 arc90 79.32,48.37 79.32,48.93 arc-90 79.57,49.18 79.58,49.18 arc-90 79.83,48.93 79.83,48.37 arc90 80.08,48.12 80.08,48.12 arc90 80.33,48.37 80.33,48.93 arc-90 80.59,49.18 80.59,49.18 arc-90 80.84,48.93 80.84,48.37 arc90 81.09,48.12 81.1,48.12 arc90 81.35,48.37 81.35,48.4 arc-90 81.6,48.65 R85.1
N$117  (via drill 0.15 layers 1-2)
  Top 0.127: IC7.R5 69.21,37.99 v69.6,37.6 | RN10.3 v74.6,42.6
  Route2 0.127: v69.6,37.6 70.2,37.6 71,38.4 71.8,38.4 74.6,41.2 v74.6,42.6
N$118  (via drill 0.15 layers 1-2)
  Top 0.127: IC7.R4 v70.4,38.4 | RN10.2 v75,43
  Route2 0.127: v70.4,38.4 70.8,38.8 71.6,38.8 74.2,41.4 74.2,42.8 74.4,43 v75,43
N$119  (via drill 0.15 layers 1-2)
  Top 0.127: IC7.R3 70.81,37.99 v71.2,37.6 | v75,40.4 RN9.1
  Route2 0.127: v71.2,37.6 72.2,37.6 v75,40.4
N$120  (via drill 0.15 layers 1-2)
  Top 0.127: IC7.P4 70.01,37.19 v70.4,36.8 | RN9.2 75.2,40 v75,39.8
  Route2 0.127: v70.4,36.8 70.8,37.2 72.4,37.2 v75,39.8
N$121  (via drill 0.15 layers 1-2)
  Top 0.127: IC7.R6 68.41,37.99 v68.8,37.6 | RN10.4 v75,42.2
  Route2 0.127: v68.8,37.6 69.2,37.2 70.2,37.2 71,38 72,38 75,41 v75,42.2
N$122  (via drill 0.15 layers 1-2)
  Top 0.127: IC7.U3 v71.6,40.4 | v75,44 75.2,44.2 R89.1
  Route2 0.127: v71.6,40.4 72,40.4 73.4,41.8 73.4,42.8 74.6,44 v75,44
N$123
  Bottom 0.254: C84.1 48.6,41.27 D2.3
  Bottom 0.406: U3.1 51.95,38.45 51.6,38.8 50.2,38.8 | 50.2,38.8 49.05,38.8 C84.1 | U3.3 50.05,38.65 50.2,38.8 | D2.3 45.29,43.01 R128.2
N$127  (via drill 0.5)
  Top 0.406: U1.4 42.77,53.55 v42.8,53.58 | R91.2 C89.1 v42.8,44.69 C88.2 R90.1
  Route3 0.406: v42.8,53.58 v42.8,44.69
N$128  (via drill 0.25)
  Top 0.406: v67.5,63.58 67.5,62.34 U2.4 | R92.1 C91.2 v67.5,54.38 C90.1 R93.2
  Route3 0.406: v67.5,54.38 v67.5,63.58
N$129
  Top 0.61: U1.5 41.66,50.41 L4.P$1
N$130
  Top 0.305: LR6.1 40.2,43.38 R90.2
  Top 0.61: R90.2 C88.1 40.24,45.84 C95.1 C96.1 39.31,48.5 38.23,49.59 L4.P$2
N$131
  Top 0.61: U2.5 66.36,60.41 L3.P$1
N$132
  Top 0.406: R92.2 64.94,51.65 LR5.1
  Top 0.61: L3.P$2 62.92,59.27 63.69,58.5 C94.1 C92.1 64.94,55.84 C91.1 R92.2
N$138  (via drill 0.15 layers 1-2, 0.15 layers 15-16, 0.25 layers 2-15)
  Top 0.127: IC7.F4 70.01,30.81 v70.4,31.2
  Route2 0.127: v70.4,31.2 v70.8,30.8
  Route15 0.127: v71.6,29.4 71.6,30 v70.8,30.8
  Bottom 0.127: R105.2 71.53,29.33 v71.6,29.4
N$140  (via drill 0.15 pad 0.1 layers 1-2, 0.25, 0.25 layers 2-15)
  Top 0.127: IC7.N16 60.39,36.39 v60,36
  Route2 0.127: v60,36 59.6,36.4 58.6,36.4 57.8,37.2 56.8,37.2 v56.4,37.6
  Route3 0.127: v56.4,37.6 56.4,51 v56.8,51.4
  Bottom 0.127: v56.8,51.4 R108.1 R106.2
N$141  (via drill 0.15 pad 0.1 layers 1-2, 0.25, 0.25 layers 2-15)
  Top 0.127: IC7.N17 59.59,36.39 v59.2,36.8
  Route2 0.127: v59.2,36.8 58.8,36.8 58,37.6 v57.2,37.6
  Route3 0.127: v57.2,37.6 56.8,38 56.8,50.2 v58,51.4
  Bottom 0.127: v58,51.4 R109.1 R107.2
N$142  (via drill 0.15 pad 0.1 layers 1-2, 0.25)
  Top 0.127: IC7.H18 58.8,32.4 v58.4,32.8
  Route2 0.127: v58.4,32.8 v57,32.8
  Bottom 0.127: v57,32.8 R110.1
N$143  (via drill 0.15 pad 0.1 layers 1-2, 0.25)
  Top 0.127: IC7.J15 61.2,33.2 v60.8,33.6
  Route2 0.127: v60.8,33.6 60.4,34 59.8,34 59,34.8 v55.6,34.8
  Bottom 0.127: R111.1 v55.6,34.8
N$144  (via drill 0.15 pad 0.1 layers 1-2, 0.25)
  Top 0.127: IC7.C3 | IC7.C3 v71.2,28
  Route2 0.127: v71.2,28 72,27.2 v72,22
  Bottom 0.127: v72,22 72,19.85 R112.1
N$146  (via drill 0.15 pad 0.1 layers 1-2, 0.25)
  Top 0.127: IC7.C6 68.39,28.41 v68.8,28
  Route2 0.127: v68.8,28 68.4,27.6 68.4,27.4 68,27 68,21.4 v68.4,21
  Bottom 0.127: v68.4,21 68.4,19.85 R113.1
N$154
  Bottom 0.406: J1.2 12.4,45.95 B1.+
N$155  (via drill 0.25, 0.25 layers 2-15)
  Route3 0.254: v37.2,46.8 36.4,47.6 35.4,47.6 34.6,46.8 24.4,46.8 24,47.2 22.8,47.2 21.4,48.6 14.62,48.6 J1.1
  Route14 0.254: v44.6,47.2 44.2,46.8 v37.2,46.8
  Bottom 0.254: R128.1 v44.6,47.2
  Bottom 0.406: D2.1 44.81,45.21 R128.1
N$156
  Bottom 0.254: R130.2 78.5,17.5 | 78.5,17.5 R129.1 | IC4.7 78.08,15.32 78.5,15.75 78.5,17.5
N$159
  Top 0.254: IC11.29 92.14,20.99 R137.2
N$160
  Top 0.254: IC11.31 90.37,23.88
  Top 0.305: 90.37,23.88 R138.2
N$161  (via drill 0.15 layers 1-2, 0.25, 0.25 layers 2-15)
  Top 0.15: IC11.3 84.71,20.49 v84.4,20.8 | v80.2,26 D3.1
  Route2 0.15: v84.4,20.8 v84,21.2 | v79.4,26 v80.2,26
  Route3 0.127: 81.95,23.25 80.93,23.25 v79.4,24.78
  Route3 0.15: v84,21.2 81.95,23.25 | v79.4,26 v79.4,24.78
  Bottom 0.127: v79.4,24.78 79.4,24.05 D11.1
N$162
  Top 0.254: IC11.28 92.36,20.49 R136.2
N$163
  Top 0.254: IC11.22 92.31,17.49 D4.1
N$164  (via drill 0.25)
  Top 0.254: LED6.A 13.49,59.15 v12.7,59.94
  Bottom 0.305: v12.7,59.94 R139.1
N$165  (via drill 0.15 layers 1-2, 0.25, 0.25 layers 2-15)
  Top 0.127: IC11.34 88.87,22.93 v88.8,23
  Route2 0.127: v88.8,23 v88.2,23
  Route3 0.127: v88.2,23 87.6,23 85,20.4 81.4,20.4 79,22.8 v78.4,22.8 | v60.6,22.8 v57.6,22.8 | v12.8,56.4 12.8,55.2 13.6,54.4 26,54.4 v29,51.4 | v38.4,39.6 39.2,38.8 v39.2,22.8
  Route14 0.127: v78.4,22.8 v60.6,22.8 | v57.6,22.8 v39.2,22.8 | v29,51.4 29.2,51.2 29.2,41.8 31.4,39.6 v38.4,39.6
  Bottom 0.127: R139.2 12.7,56.5 v12.8,56.4
N$166
  Top 0.254: IC11.37 87.37,27.17 J_TP2.TP
N$167
  Top 0.254: IC11.36 87.87,26.07 J_TP1.TP
N$168
  Top 0.254: IC11.5 Q12.3 82.6,18.35 C103.2
N$169
  Top 0.254: 86.87,15.63 87.3,15.2 87.3,14.85 C117.2 | L12.2 86.3,15 86.3,15.2 86.83,15.73 86.87,15.63 | IC11.13 86.87,15.63
N$170
  Top 0.5: C117.1 88.85,13.52 L13.1
N$172  (via drill 0.25)
  Top 0.254: R148.1 53.85,6.55 53.6,6.8 v53.6,7.2
  Bottom 0.406: v53.6,7.2 52.8,8 50.4,8 49.2,6.8 49.2,5.7 C6.1
  Bottom 0.61: L15.2 46.75,7.2 | 46.75,7.2 46.75,5.7 C4.1 C6.1 | 43.2,7.05 46.6,7.05 46.75,7.2 | U5.6 43.45,6.8 43.2,7.05 | 43.2,7.05 41.7,7.05 C123.1 41.2,7.15 C124.1
N$173
  Top 0.305: IC12.8 14.45,35.5 R141.2
N$175
  Top 0.305: IC12.2 8.85,36 C119.1
N$177
  Bottom 0.254: R145.1 46.03,14 USB.3
N$178
  Bottom 0.254: R146.1 46.03,12 USB.2
N$179  (via drill 0.25)
  Top 0.254: IC13.16 53.35,11.75 v53,11.4
  Bottom 0.254: R145.2 50.1,15.15 D9.2 54.05,15.15 54.4,14.8 54.4,13.6 53.6,12.8 53.6,12 v53,11.4
N$180  (via drill 0.25)
  Top 0.254: IC13.15 53.05,12.25 v53,12.2
  Bottom 0.254: R146.2 50.35,12 D8.2 51.85,12.2 v53,12.2
N$182
  Top 0.254: IC13.21 55.75,8 C128.1
N$183
  Top 0.254: IC13.7 57.25,15.5 57.75,16 58.25,16 58.5,16.25 C125.1
N$184
  Top 0.254: IC13.22 56.25,8.95 56.8,8.4 56.8,7 56.4,6.6 55.95,6.6 C128.2
N$186
  Bottom 0.305: U5.5 42.5,4.7 42.1,4.3 39.75,4.3 C126.1
N$187
  Top 0.254: IC13.11 55.25,14.75 55,15 54,15 53.25,14.25 R150.2
N$188
  Top 0.254: IC13.10 55.75,15.25 55.5,15.5 52.7,15.5 R151.2
OVRCNT_B  (via drill 0.15 pad 0.1 layers 1-2, 0.25 layers 2-15, 0.25 pad 0.1)
  Top 0.127: IC7.C14 v61.6,28
  Route2 0.127: v55.2,26.4 60.2,26.4 60.8,27 60.8,27.6 61.2,28 v61.6,28
  Route3 0.127: v40.7,5.5 41.8,4.4 46.2,4.4 50,8.2 v50,26.4
  Route14 0.127: v55.2,26.4 v50,26.4
  Bottom 0.15: U5.4 v40.7,5.5
PGOOD  (via drill 0.25)
  Top 0.305: IC12.9 13,36 v13.4,36.4 | v12.6,31.4 13.39,31.4 R142.1
  Route14 0.305: v13.4,36.4 12.6,35.6 v12.6,31.4
POWER_ON  (via drill 0.25, 0.25 layers 2-15)
  Top 0.254: U4.3 18.86,25.94 v19.2,25.6 | v46.7,52.4 45.46,52.4
  Top 0.305: v14.8,30.2 14.75,30.25 R142.2 R94.1 14.8,32.72 v14.8,33.6 | v9.6,21 9.6,21.68 IC5.5 | 45.46,52.4 U1.3 | v70.4,63.2 70.4,62.64 U2.3
  Route3 0.254: v33.6,42.4 23.6,42.4 v14.8,33.6 | v50.4,52.4 59.6,52.4 v66.4,59.2 | v33.6,49.2 36.8,52.4 39.9,52.4 42.1,54.6 44.5,54.6 v46.7,52.4 | v19.2,25.6 14.8,25.6
  Route3 0.305: v14.8,30.2 14.8,25.6 14.8,24.8 11,21 v9.6,21
  Route14 0.254: v33.6,42.4 v33.6,49.2 | v66.4,59.2 v70.4,63.2 | v50.4,52.4 v46.7,52.4
RDN  (via drill 0.25)
  Route3 0.254: v31.75,23 31.75,19.55 30.55,18.35 29.2,18.35 ETH.2
  Bottom 0.254: U201.11 33.88,25.63 33,24.75 33,24 32.5,23.5 32.5,23.25 32.25,23 v31.75,23 R6.1
RDP  (via drill 0.25)
  Route3 0.254: v31.75,24.25 32,24.25 32.3,23.95 32.3,18.85 31.75,18.3 31.75,16.55 31.2,16 28.11,16 ETH.1
  Bottom 0.254: U201.12 33.63,26.13 32.5,25 32.5,24.5 32.25,24.25 v31.75,24.25 R5.1
RFBOUT  (via drill 0.25)
  Route14 0.254: v33,28.25 33.5,28.75 v33.5,29.75 33.5,31.9 v33.85,32.25 34.05,32.45 39.55,32.45 39.8,32.2 v41.2,32.2
  Bottom 0.254: U201.19 33.62,29.63 v33.5,29.75 | C131.1 41.4,32.6 41.2,32.4 v41.2,32.2 40.2,31.2 40,31.2 39.62,30.82 U201.30 | U201.16 33.12,28.13 v33,28.25
  Bottom 0.256: C133.1 30.99,33.41 32,32.4 33.7,32.4 v33.85,32.25
  Bottom 0.305: C132.1 32.75,28 v33,28.25
SPEED  (via drill 0.15 pad 0.1 layers 1-2, 0.25 layers 2-15)
  Top 0.127: IC7.A14 v61.6,26.4
  Route2 0.127: v61.6,26.4 60.8,25.6 v57.2,25.6
  Route3 0.127: ETH.C1 34.09,3.61 35.6,2.1 38.9,2.1 40,3.2 40,3.7 40.4,4.1 46.5,4.1 50.4,8 v50.4,25.6
  Route14 0.127: v57.2,25.6 v50.4,25.6
SPI1_CLK/SCK0  (via drill 0.15 pad 0.1 layers 1-2, 0.25, 0.25 layers 2-15)
  Top 0.127: IC7.C9 66,28.4 v65.6,28 | 76.8,7.79 EXT.18 77,7.58 v77,9.2
  Route2 0.127: v65.6,28 65.2,27.6 65.2,27 65.6,26.6 65.6,20.2 v65.8,20
  Route14 0.127: v65.8,20 72,20 73.2,18.8 73.2,12.8 76.6,9.4 76.8,9.4 v77,9.2
SPI1_DATIN/MISO0/GPI_25  (via drill 0.15 pad 0.1 layers 1-2, 0.25, 0.25 layers 2-15)
  Top 0.127: IC7.C10 65.2,28.4 v64.8,28 | EXT.14 74.4,7.64 v74.4,9.2
  Route2 0.127: v64.8,28 64.4,27.6 64.4,27 64.8,26.6 v64.8,20
  Route14 0.127: v64.8,20 65.6,19.2 71.6,19.2 72.4,18.4 72.4,12.4 74.4,10.4 v74.4,9.2
SPI1_DATIO/MOSI0  (via drill 0.15 pad 0.1 layers 1-2, 0.25, 0.25 layers 2-15)
  Top 0.127: IC7.B9 66,27.6 v65.6,27.2 | EXT.16 75.8,7.51 v75.8,9.2
  Route2 0.127: v65.6,27.2 65.6,27 66,26.6 66,20.4 66.4,20 v66.4,19.6
  Route14 0.127: v66.4,19.6 71.8,19.6 72.8,18.6 72.8,12.6 75.8,9.6 v75.8,9.2
SPI2_CLK/SCK1/LCDVD[23]  (via drill 0.15 pad 0.1 layers 1-2, 0.25 layers 2-15, 0.25 pad 0.1)
  Top 0.127: IC7.B10 65.2,27.6 v64.8,27.2 | EXT.4 68.19,8.99 v68.4,9.2
  Route2 0.127: v64.8,27.2 64.8,27 65.2,26.6 65.2,19.2 v64.4,18.4
  Route14 0.127: v64.4,18.4 64.8,18 67.4,18 68.4,17 v68.4,9.2
SW_3V3
  Top 0.305: 8.08,35.6 8.2,35.6 8.3,35.5 IC12.3
  Top 0.61: 5.9,35.6 4.45,35.5 D7.C 4,40 2.9,41.1 L14.1 | 5.9,35.6 8.08,35.6 | C119.2 6.15,35.65 5.9,35.6
  pour Top (isolate 0.406): 2,44 6.25,44 6.25,35.5 2,35.5
SW_5V
  Top 0.305: 8.3,22.83 8.45,22.8 8.52,22.73 IC5.3
  Top 0.61: 5.8,22.83 4.45,22.73 D5.C 4,27.13 L16.1 | 5.8,22.83 8.3,22.83 | C10.2 6.15,22.88 5.8,22.83
  pour Top (isolate 0.406): 2,31 6.25,31 6.25,22.75 6.25,22.5 2,22.5
TC1
  Bottom 0.254: TC1.TP R112.2
TC2
  Bottom 0.254: TC2.TP R113.2
TDN  (via drill 0.25)
  Route3 0.254: v31.75,25.5 32.25,25.5 32.85,24.9 32.85,17.32 ETH.6
  Bottom 0.254: U201.14 33.88,27.13 32.25,25.5 v31.75,25.5 R9.1
TDP  (via drill 0.25)
  Route3 0.254: v31.71,26.75 32.25,26.75 33.4,25.6 33.4,18.75 34.3,17.85 34.3,16.6 32.75,15.05 32.24,15.05 ETH.5
  Bottom 0.254: U201.15 33.63,27.63 32.75,26.75 v31.71,26.75 R7.1
U1_RX/GPI_15  (via drill 0.15 layers 1-2, 0.25 layers 2-15)
  Top 0.127: IC7.K15 61.21,33.99 v61.6,33.6
  Top 0.254: R136.1 v94.7,20.2
  Route2 0.127: v61.6,33.6 61.2,33.2 v61.2,29.8 | v94.7,20.8 v94.7,20.2
  Route3 0.127: v91.8,25.4 92.2,25.4 93.2,24.4 93.2,22.3 v94.7,20.8
  Route14 0.127: v61.2,29.8 61.6,29.8 65,26.4 73.4,26.4 74.2,25.6 80.6,25.6 81,26 91.2,26 v91.8,25.4
U1_TX  (via drill 0.15 layers 1-2, 0.15 pad 0.1 layers 1-2, 0.25 layers 2-15)
  Top 0.127: IC7.K16 60.4,34 v60.8,34.4
  Top 0.254: R137.1 v94.7,21.5
  Route2 0.127: v94.7,22 v94.7,21.5 | v61.6,30.4 61.6,33 62,33.4 62,33.8 61.4,34.4 v60.8,34.4
  Route3 0.127: v92.6,25.6 93.6,24.6 93.6,22.5 94.1,22 v94.7,22
  Route14 0.127: v61.6,30.4 65.2,26.8 73.6,26.8 74.4,26 78.8,26 79.2,26.4 91.8,26.4 v92.6,25.6
U2_HCTS/U3_CTS/GPI_16  (via drill 0.15 pad 0.1 layers 1-2, 0.25, 0.25 layers 2-15, 0.25 pad 0.1 layers 2-15)
  Top 0.127: IC7.J18 58.8,33.2 v58.4,33.6 | v70.8,9.2 70.8,7.58 EXT.8
  Route2 0.127: v58.4,33.6 v55.6,33.6
  Route3 0.127: v55.6,33.6 55.6,33.2 54.2,31.8 54.2,24 63.4,14.8 v70,14.8
  Route14 0.127: v70,14.8 70,10.6 70.8,9.8 v70.8,9.2
U3_RX/GPI_18  (via drill 0.15 layers 1-2, 0.25, 0.25 layers 2-15)
  Top 0.127: IC7.J14 61.6,32.8 61.6,32.2 61.8,32 v62.4,32 | v70.8,5.4 70.8,3.77 EXT.7
  Route2 0.127: v62.4,32 62.4,31.2 v62,30.8 | v63.6,25.6 v63.6,19.6
  Route14 0.127: v62,30.8 61.4,30.8 60.8,30.2 60.8,29.6 63.2,27.2 63.2,26 v63.6,25.6 | v63.6,19.6 64.2,19 64.6,19 65.2,18.4 68,18.4 69.6,16.8 69.6,10.4 70.4,9.6 70.4,5.8 v70.8,5.4
U3_TX  (via drill 0.15 pad 0.1 layers 1-2, 0.25, 0.25 layers 2-15, 0.25 pad 0.1 layers 2-15)
  Top 0.127: IC7.J17 59.6,33.2 v59.2,33.6 | v69.6,5.4 69.6,3.83 EXT.5
  Route2 0.127: v59.2,33.6 58.8,34 v55.2,34
  Route3 0.127: v55.2,34 55.2,33.4 53.8,32 53.8,23.8 63.2,14.4 v69.2,14.4
  Route14 0.127: v69.2,14.4 69.2,10.2 70,9.4 70,5.8 v69.6,5.4
U5_RX/GPI_20  (via drill 0.15 pad 0.1 layers 1-2, 0.25, 0.25 layers 2-15)
  Top 0.127: IC7.F18 v58.19,30.81 v58.2,30.8 | UART5.4 26.65,39.25 v26.6,39.2
  Route2 0.127: v58.2,30.8 v56.8,30.8
  Route3 0.127: v45.2,36.8 v45.2,31.2
  Route14 0.127: v45.2,36.8 30,36.8 27.6,39.2 v26.6,39.2 | v45.2,31.2 47.2,31.2 47.6,30.8 v56.8,30.8
U5_TX  (via drill 0.15 pad 0.1 layers 1-2, 0.25, 0.25 layers 2-15)
  Top 0.127: IC7.H15 v60.8,32.8 | UART5.5 25.07,38.73 v25.2,38.6
  Route2 0.127: v60.8,32.8 60.4,32.4 v57.6,32.4
  Route3 0.127: v44.4,36.4 v44.4,32.4
  Route14 0.127: v44.4,36.4 29.8,36.4 27.6,38.6 v25.2,38.6 | v57.6,32.4 v44.4,32.4
USB_DAT_VP  (via drill 0.15 pad 0.1 layers 1-2, 0.25, 0.25 layers 2-15)
  Top 0.127: IC7.D5 v69.6,28.8 | 53.95,12.8 IC13.14
  Top 0.15: IC13.14 53.25,12.75 v53,13 52.8,13 52.5,12.7 52.5,12.1 52.15,11.75 R152.2
  Route2 0.127: v69.6,28.8 69.2,28.4 69.2,27 68.8,26.6 v68.8,22
  Route14 0.127: v68.8,22 62.2,22 55.4,15.2 55.4,14.15
  Route14 0.15: v53,13 54.25,13 55.4,14.15
USB_I2C_SCL  (via drill 0.15 layers 1-2, 0.25, 0.25 layers 2-15)
  Top 0.127: IC7.E5 | IC7.E5 v69.6,29.6 | 60.55,11.75 v60.6,11.8 60.65,11.75
  Top 0.254: IC13.3 60.55,11.75 | R143.1 60.65,11.75
  Route2 0.127: v69.6,29.6 68,28 68,27.6 67.6,27.2 v67.6,20.4
  Route14 0.127: v67.6,20.4 63.4,20.4 60.6,17.6 v60.6,11.8
USB_I2C_SDA  (via drill 0.15 layers 1-2, 0.25, 0.25 layers 2-15)
  Top 0.127: IC7.E6 v68.8,29.6 | 59.95,11.25 v60,11.2
  Top 0.254: IC13.2 59.95,11.25 | R144.1 60.7,10.5 v60,11.2
  Route2 0.127: v66.8,20.8 66.8,29 67,29.2 68.4,29.2 v68.8,29.6
  Route14 0.127: v66.8,20.8 63.2,20.8 60.2,17.8 60.2,11.4 v60,11.2
USB_SE0_VM  (via drill 0.15 layers 1-2, 0.15 pad 0.1 layers 1-2, 0.25 layers 2-15)
  Top 0.127: IC7.C5 v69.6,28
  Top 0.15: IC13.13 v54,14
  Top 0.254: R153.2 52.2,13 52.8,13.6 53.65,13.6 IC13.13
  Route2 0.127: v69.6,28 69.6,23 70,22.6 v70,22.4
  Route2 0.15: v54,14 v54.8,14.8
  Route14 0.127: v70,22.4 62,22.4 54.8,15.2 v54.8,14.8
USB_SHIELD
  Route3 0.61: USB.P$6 48.5,9.3 47.2,8 44.58,8 USB.P$5
  Bottom 0.406: RC21.1 43.28,18.6 USB.P$7 | R34.2 48.72,18.6 USB.P$8
  pour Top: 43.2,0 43.2,16.8 48.8,16.8 48.8,0
USB_VBUS_CTRL  (via drill 0.25)
  Top 0.254: IC13.1 58.85,10.75 v60,9.6 60.35,9.25 R149.1 R8.2
  Route3 0.127: 58.4,8 51.1,8 46.8,3.7 40.9,3.7 v40.6,3.4
  Route3 0.15: 58.4,8 v60,9.6
  Bottom 0.254: U5.3 41.1,2.9 v40.6,3.4
VB_DIG
  Top 0.254: IC11.35 88.37,23.37 C116.1
VB_RAM
  Top 0.254: IC11.25 92.56,18.99 C115.1
VB_RF  (via drill 0.15 layers 1-2)
  Top 0.15: IC11.14 87.37,16.83 87.2,17 86.5,17 86.4,16.9 86.4,16.3
  Top 0.254: C113.1 84.6,14.7 84.6,14.8 85.5,15.7 v86.2,15.7 86.37,15.87 IC11.12 | 86,11.63 C114.1 | IC11.14 87.37,15.78 v87.45,15.7
  Top 0.35: C113.1 L12.1
  Top 0.5: L12.1 86,11.63
  Route2 0.254: v86.2,15.7 v87.45,15.7
VB_SYNTH
  Top 0.254: IC11.6 84.19,18.99 83.9,18.7 83.9,18.2 82.9,17.2 81.9,17.2 81.6,16.9 80.95,16.9 C111.1
VB_VCO
  Top 0.254: IC11.8 84.39,17.99 83.2,16.8 82.2,16.8 81.9,16.5 81.9,16.05 C112.1
VDD_1V2  (via drill 0.15 layers 1-2, 0.15 layers 15-16, 0.25, 0.25 layers 2-15)
  Top 0.127: IC7.R17 v60,37.6 | IC7.L12 v64,35.2 | IC7.T18 v59.2,38.4 | IC7.T16 60.38,38.78 v60,38.4 | IC7.P15 v60.8,36.8 | IC7.M13 v63.2,36
  Top 0.305: LR6.2 42.5,42.1 v42.8,42.4
  Top 0.406: v42.8,42.4 v42.8,41.6 v43.6,41.6 v43.6,42.4 v42.8,42.4
  Route2 0.127: v59.2,38.4 v58.8,38.8 | v59.6,38.8 v60,38.4 | v62.8,35.6 v63.2,36 | v60.8,36.8 v60.4,36.4 | v60,37.6 v59.6,38
  Route2 0.15: v64,35.2 v64,34.4
  Route14 0.305: v64,34.4 v62.8,35.6 62.8,36.4 63.2,36.8 | v60.4,36.4 59.6,37.2 v59.6,38 | v59.6,38 v59.6,38.8 | v58.8,38.8 v59.6,38.8 | v59.6,38 v60,37.6 60.8,37.6 IC7.P15 | v59.6,38.8 59.6,40.4 58.4,41.6 50.4,41.6 49.6,42.4 | 61.6,36.8 IC7.P15 | IC7.P15 v62,38 62.8,38 63.2,37.6 63.2,36.8 | 63.2,36.8 v64,36
  Route14 0.406: 49.6,42.4 v43.6,42.4
  Route15 0.127: v58.2,38.8 v58.8,38.8 | v58.2,40 58.4,40 v59.6,38.8 | v58.2,37.6 58.4,37.6 58.8,38 v59.6,38 | v58.2,36.4 v60.4,36.4 59.6,37.2 58.6,37.2 v58.4,37 | v64.4,35.6 v64,36 | v62,38 v61.6,38.4
  Bottom 0.127: R47.2 64.4,35.4 v64.4,35.6 | C39.1 C40.1 60.85,38.4 v61.6,38.4 | v58.4,37 58.8,36.6 R46.2 | C48.1 57.4,40.8 v58.2,40 | C49.1 57.4,39.6 v58.2,38.8 | C47.1 57.4,38.4 v58.2,37.6 | C46.1 57.4,37.2 v58.2,36.4
  pour Route14: 58.4,43.2 63.8,37.8 63.8,36.2 64.4,35.6 64.4,35 63.8,34.4 63.4,34.4 62.8,35 61,35 55.2,40.8 42.6,40.8 42,41.4 42,42.8 42.4,43.2
VDD_1V2_RTC  (via drill 0.15 layers 1-2, 0.15 layers 15-16, 0.25, 0.25 layers 2-15)
  Top 0.127: IC7.N15 v61.19,36.39 v60.8,36 | IC7.L13 62.8,34.8 v62.4,34.4
  Route2 0.127: v60.8,36 v61.2,36.4 | v62.4,34.4 v62.8,34
  Route3 0.254: v57,36.4 56.6,36.4 55.8,37.2 55.8,39 v54.8,40
  Route15 0.127: v61.2,36.4 60.4,35.6 59.6,35.6 59.2,35.2 v58.6,35.2 | v62.8,34 v58.8,34
  Bottom 0.127: v58.6,35.2 58.05,35.2 C43.1
  Bottom 0.254: v54.8,40 54.15,40 C85.1 | U3.5 51.95,42.4 R56.2
  Bottom 0.305: R48.2 v58.8,34 58.6,34.2 C44.1 C43.1 57.85,36.15 57.6,36.4 v57,36.4
  Bottom 0.406: U3.5 52.55,40.1 C85.1
VDD_1V2_VAR(1V33)  (via drill 0.15 layers 1-2, 0.15 layers 15-16, 0.25, 0.25 layers 2-15)
  Top 0.127: IC7.M11 v64.8,35.2 | IC7.M7 | IC7.M7 v67.2,35.2 | IC7.J7 v67.2,33.6 | v67.2,32 | v67.2,32 IC7.G7 | IC7.G9 v66,32.2 | IC7.J12 v64.2,33.2 | IC7.G11 v64.8,32
  Top 0.406: LR8.2 25.63,33.63 v25.4,33.4 | v25.4,33.4 v26.2,33.4 v26.2,32.6 v25.4,32.6 v25.4,33.4
  Route2 0.127: v64.2,33.2 v65.2,33.2 | v64.8,32 v64.4,32.4 | v66,32.2 66,32.6 v65.8,32.8 | v66.8,32.4 v67.2,32 | v66.8,33.2 v67.2,33.6 | v66.8,34.8 v67.2,35.2 | v64.8,34.6 v64.8,35.2
  Route14 0.406: v66.8,34.8 66.6,34.6 v64.8,34.6 65.2,34.2 v65.2,33.2 65.6,32.8 v65.8,32.8 | v65.8,32.8 66.4,32.8 | 66.4,32.8 v66.8,33.2 | 66.4,32.8 v66.8,32.4 | v65.8,32.8 65.4,32.4 v64.4,32.4 63.6,32.4 61.6,34.4 60.2,34.4 57.6,37 46.6,37 44,34.4 26.4,34.4 v25.4,33.4
  Route15 0.127: v64.8,32.8 v64.4,32.4 | v64.8,34 64.8,33.6 v65.2,33.2 | v66.8,34.8 v67.6,34 | v66.6,34 66.6,33.4 v66.8,33.2 | v68,31.4 67.8,31.4 v66.8,32.4 | v64.8,31.2 64.8,31.8 v65.8,32.8 | v65.6,34 65.4,34 v64.8,34.6
  Bottom 0.127: C33.1 v65.6,34 | C32.1 66.8,34.2 v66.6,34 | C31.1 68,34.4 v67.6,34 | C36.1 v64.8,34 | C37.1 v64.8,32.8 | C38.1 64.6,31 v64.8,31.2 | C35.1 v68,31.4
  pour Route14: 57.8,37.4 60.6,34.6 62.6,34.6 63.2,34 64.2,34 65,34.8 66.6,34.8 67,34.4 67,32.6 67.2,32.4 67.8,32.4 67.8,31 64.6,31 62.8,32.8 59.4,32.8 56.4,35.8 46.8,35.8 45,34 30,34 27.8,31.8 25.2,31.8 24.2,32.8 24.2,34.6 25.2,35.6 43.8,35.6 45.6,37.4
VDD_3V3  (via drill 0.15 layers 1-2, 0.15 layers 15-16, 0.25, 0.25 layers 2-15, 0.38, 0.5)
  Top 0.127: 66,30.8 IC7.F9 v66.4,30.4 | IC7.F13 v62.81,30.79 v62.4,30.4 | IC7.J13 v63.2,33.6 | IC7.F8 v67.2,30.4 | IC7.F7 v68,30.4 | IC7.G6 v68.8,31.2 | IC7.J5 v69.6,32.8 | IC7.H6 v68.4,32.4 v68.8,32 | IC7.H13 v63.2,32.8
  Top 0.254: JTAG.1 19.34,51.74 v19.4,51.8
  Top 0.305: IC12.1 9.65,36.85 9.5,37 | 13,34.5 IC12.6 | R94.2 13.45,34.45 v13.5,34.5
  Top 0.406: v13.5,34.5 13,34.5 | EXT.11 EXT.9 | v70.2,57.2 70.2,58.45 C87.1 | L11.2 83.25,25.35 v82.5,24.6 | L5.1 52.75,19.85 v52.6,20 | JUART1.4 103.36,26.95 101.9,26.95 v101.8,27.05
  Top 0.61: 9.5,37 9.5,37.5 v10,38 10,41.5 | 10,41.5 L14.2 | 10,41.5 11.1,41.5 C121.1 | U1.1 45.55,50.23 C86.1 45.85,48.8 v46.8,48.8 | C87.1 70.25,60.23 U2.1 | U4.1 18.68,28.57 C97.1 18.68,30.68 v19.2,31.2 | v46.8,48.8 v47.6,48.8 v47.6,49.6 | EXT.9 v72,5.6 v72.8,5.6 | v82.5,24.6 v81.7,24.6 | v46.8,49.6 v46.8,48.8 | v19.2,31.2 v18.4,31.2 v18.4,32 v19.2,32 v19.2,31.2 | v71,57.2 v70.2,57.2 v70.2,56.4 v71,56.4 v71,57.2
  Route2 0.127: v68,30.4 v68,29.8 | v67.2,30.4 v66.8,30 | v66.4,30.4 v66,30 | v62.4,30.4 v62.8,30.8 | v63.2,32 v62.8,31.6 | v69.6,32.8 v70,32.4 | v68.8,31.2 v69.2,31.6 | v68.8,32 v68.4,32.4 | IC7.J13 v63.2,33.6 v63.2,32.8 IC7.H13
  Route14 0.254: v70,32.4 69.8,32.4 69.2,31.8 v69.2,31.6 | v71,57.2 v70.2,57.2 v70.2,56.4 v71,56.4 | v46.8,49.6 v46.8,48.8 | v47.6,49.6 v47.6,48.8 | v27,49.6 26.6,49.6 26.2,50 26.2,50.8 v27,51.6 27,52.2 26.4,52.8 | 32.8,52.8 32.8,54.2 v32.4,54.6
  Route14 0.305: v68.4,32.4 IC7.G6 v69.19,31.61 | v27,29.6 27,23.8 26.4,23.2 | v69.19,31.61 v69.2,31.6 | v69.19,31.61 69.19,30.79 v68.8,30.4 68.2,29.8 v68,29.8 67,29.8 v66.8,30 v66,30 65.2,30 64.6,29.4 v63.8,29.4 63.6,29.6 63.6,30 v62.8,30.8 v62.8,31.6 v62.81,31.61 IC7.H13
  Route14 0.406: 32.8,52.8 36.4,56.4 v38,56.4 v47,56.4 v56.4,56.4 v58,56.4 69.4,56.4 v70.2,57.2 | v50.2,47 48.4,48.8 v47.6,48.8 47.8,48.6 v47.8,46.8 | v38.8,47.8 38.8,48.4 38.4,48.8 | v62.8,31.6 61.2,31.6 59.2,29.6 | v27,29.6 30.4,33 v32.6,33 41.4,33 43.2,31.2 v44.4,31.2
  Route14 0.61: 15,43 v11,43 10.8,42.8 10.8,39 10,38.2 v10,38 | 15,43 16.8,44.8 16.8,51.8 17.8,52.8 19.2,52.8 | 19.2,52.8 26.4,52.8 32.8,52.8 36.8,48.8 38.4,48.8 v46.8,48.8 v47.6,48.8 | 15,43 17,41 17,31.2 | 17,31.2 17,26.2 20,23.2 26.4,23.2 v27.2,23.2 29.6,23.2 31.2,21.6 36.8,21.6 37.6,20.8 v44,20.8 47.2,20.8 48,20 51.2,20 | 51.2,20 v52.6,20 56.8,20 59.2,22.4 59.2,24.8 | 59.2,29.6 59.2,24.8 | v19.2,31.2 17,31.2 | 59.2,24.8 72.8,24.8 73.6,24 79.8,24 | v94.4,42.8 v95.2,42.8 95.6,42.8 96.8,41.6 96.8,28.4 v92.4,24 v91.4,24 88,24 87.4,24.6 v82.5,24.6 v81.7,24.6 81.1,24 79.8,24 | v19.4,51.8 19.4,52.6 19.2,52.8 | 51.2,20 52,19.2 52,11.2 52.8,10.4 62.4,10.4 64.2,8.6 v64.2,7.6 64.2,6.8 66.4,4.6 71.6,4.6 72,5 v72,5.6 | v77.75,13.75 77.75,16 v77.5,16.25 77.4,16.35 77.4,18.8 78.2,19.6 79.2,20.5 79.8,21.1 79.8,24 | 96.75,28.4 100.45,28.4 v101.8,27.05
  Route15 0.127: v62.8,31.6 v60.4,31.6 | v62.8,30.8 62,30 v62,29.6 | v66,30 v66,29.2 | v66.8,30 v66.8,29.2 | v68.4,29.4 v68,29.8 67.6,29.4 v67.6,29.2 | v68,32.8 v68.4,32.4 | v69.2,30 v68.8,30.4 | IC7.H13 v60.4,32.4 | v63.8,29.4 63.4,29.4 v63.2,29.6
  Bottom 0.127: v60.4,31.6 60.25,31.6 C50.1 | v62,29.6 C59.1 | C54.1 v68,32.8 | v60.4,32.4 C51.1 | v63.2,29.6 63.2,29.05 C58.1 | v66,29.2 66,28.65 C56.1 | v66.8,29.2 66.8,28.85 C57.1 | v68.4,29.4 68.4,28.65 C52.1 | C53.1 70,29.2 v69.2,30 | C55.1 67.05,29.75 v67.6,29.2
  Bottom 0.254: C67.1 92.25,18.9 IC9.12 92.25,23.85 v92.4,24 | IC9.37 92.25,41.5 92.75,42 92.75,42.52 C68.1 | R74.2 R73.2 | R12.1 52.6,45.45 | 52.6,45.45 C66.1 | IC8.5 52.95,45.1 52.6,45.45 | R131.2 56.52,56.52 v56.4,56.4 | R21.2 v27,51.6 | v27,49.6 26.6,49.2 R23.2 R20.2 | R22.2 17.15,44.05 v17.2,44 | v32.4,54.6 32.4,54.4 32,54 31.45,54 R18.2 | D1.1 60.5,50.1 v60.4,50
